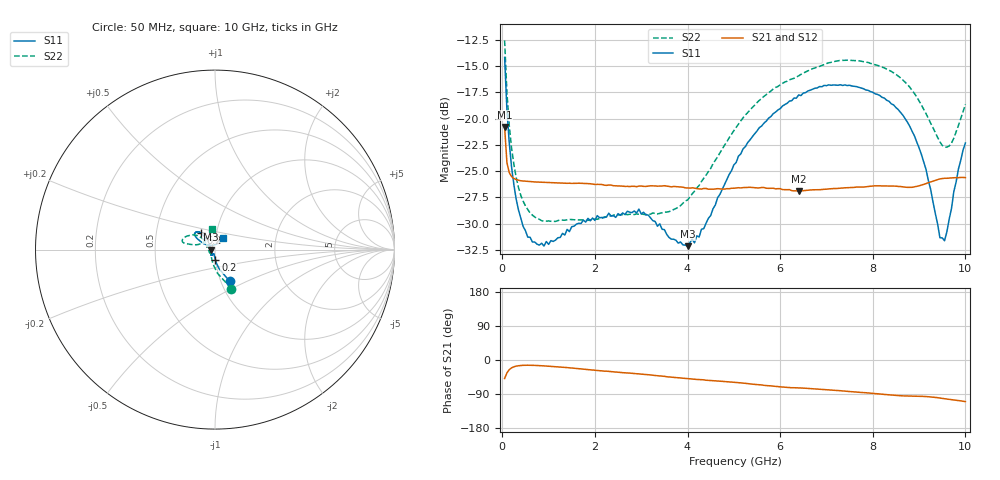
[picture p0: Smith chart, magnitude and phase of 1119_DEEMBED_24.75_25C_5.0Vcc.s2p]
!Hittite Microwave Corp.
!Digital Attenuator/PhaseShifter Rev 1.4.0
!Filename: C:\DATA\DATA\1119_DEEMBED_24.75_25C_5.0Vcc.s2p
!VNA ID: Agilent Technologies,N5224A,MY51441122,A.10.45.03
!Device type:
!2 Port Calibration.
!Temp(C): 25
!Lot Number:
!Serial Number:
!Operator:
!Misc:
!Attenuator:  24.750
# GHZ S DB R 50.0
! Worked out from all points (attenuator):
!   200 points, 50 MHz to 10 GHz, reference 50 ohm
!   highest |S21| = -20.80 dB at 50 MHz (marker M1); lowest = -26.9 dB at 6.4 GHz (marker M2)
!   lowest |S11| = -32.1 dB at 4 GHz (marker M3), VSWR 1.05, Z = 47.6 - j0.0234 ohm
!   |S11| at or under -10 dB: start of sweep to end of sweep
!   |S22| runs from -29.8 to -12.6 dB; largest |S21 - S12| = 0.00017
!   S11 on the Smith chart (normalised r, x): 50 MHz: 1.10, -0.41; 200 MHz: 1.00, -0.12; 6.2 GHz: 0.84, +0.16; 10 GHz: 1.08, +0.14
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0.05  -14.17 -65.1  -20.80 -48.8  -20.81 -48.9  -12.55 -67.3
0.1  -19.18 -77.7  -24.19 -34.0  -24.18 -34.0  -17.51 -83.8
0.2  -24.59 -87.3  -25.52 -20.8  -25.51 -20.7  -22.79 -100.5
0.35  -28.70 -93.8  -25.87 -15.1  -25.87 -15.1  -26.57 -114.5
0.65  -31.75 -103.6  -26.02 -14.0  -26.01 -14.0  -29.19 -130.0
1.75  -29.67 -120.0  -26.18 -24.0  -26.18 -24.1  -29.65 -140.6
2.95  -28.62 -125.2  -26.42 -36.6  -26.43 -36.6  -29.10 -159.8
3.4  -30.02 -140.4  -26.43 -41.9  -26.43 -41.9  -29.02 -173.4
4  -32.15 -179.4  -26.61 -49.2  -26.62 -49.3  -27.75 162.3
4.25  -31.28 160.9  -26.69 -51.8  -26.71 -51.8  -26.37 152.5
5.05  -24.18 131.0  -26.61 -59.3  -26.62 -59.3  -20.83 138.8
6.2  -18.33 130.0  -26.76 -72.7  -26.78 -72.8  -16.30 147.2
6.4  -17.74 131.5  -26.90 -73.7  -26.92 -73.8  -15.92 150.0
6.7  -17.19 134.4  -26.78 -75.8  -26.79 -75.9  -15.24 154.0
7.5  -16.82 142.4  -26.57 -83.2  -26.57 -83.2  -14.44 163.6
8.35  -18.34 147.8  -26.42 -91.8  -26.43 -91.8  -15.38 168.1
8.9  -21.64 151.3  -26.50 -95.2  -26.51 -95.2  -17.61 167.6
9.15  -24.84 151.3  -26.19 -96.4  -26.21 -96.5  -19.52 165.3
9.45  -31.35 119.9  -25.74 -100.4  -25.75 -100.4  -22.21 149.3
9.55  -31.63 93.0  -25.68 -102.2  -25.69 -102.2  -22.70 138.1
9.7  -28.56 64.9  -25.65 -104.6  -25.66 -104.6  -22.33 119.9
10  -22.32 54.9  -25.62 -109.7  -25.63 -109.7  -18.64 98.5
